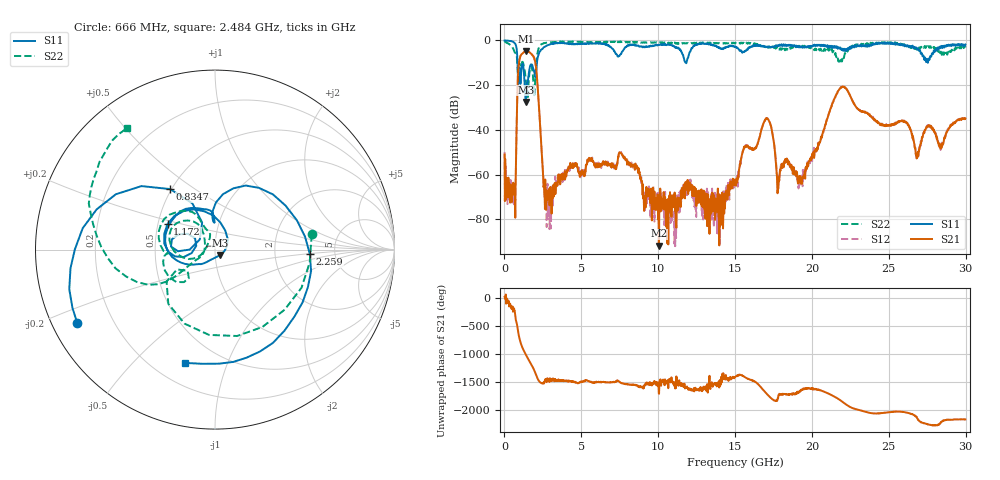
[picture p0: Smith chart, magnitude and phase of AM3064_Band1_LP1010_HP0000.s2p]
# Hz S DB R 50.0
!freq dBS11 angS11 dBS21 angS21 dBS12 angS12 dBS22 angS22
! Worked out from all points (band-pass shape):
!   1600 points, 10 MHz to 29.98 GHz, reference 50 ohm
!   highest |S21| = -4.68 dB at 1.397 GHz (marker M1); lowest = -91.9 dB at 10.04 GHz (marker M2)
!   |S21| within 3 dB of the highest: 1.011 GHz to 1.92 GHz (909.2 MHz wide, 62 % of centre)
!   lowest |S11| = -27.5 dB at 1.378 GHz (marker M3), VSWR 1.09, Z = 53 - j3.14 ohm
!   |S11| at or under -10 dB: 848.7 MHz to 2.111 GHz (1.263 GHz wide, 85.3 % of centre); 11.80178 GHz to 11.83796 GHz (36.18 MHz wide, 0.306 % of centre); 27.54303 GHz to 27.54479 GHz (1.759 MHz wide, 0.00639 % of centre)
!   |S22| runs from -26.2 to -0.3 dB; largest |S21 - S12| = 0.0077
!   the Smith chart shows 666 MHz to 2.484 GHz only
!   S11 on the Smith chart (normalised r, x): 666 MHz: 0.07, -0.25; 834.7 MHz: 0.49, +0.40; 1.172 GHz: 0.56, +0.18; 2.259 GHz: 3.23, -0.23; 2.484 GHz: 0.32, -0.72
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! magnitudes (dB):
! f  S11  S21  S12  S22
! 10 MHz  0.0  -51.1  -49.9  -0.3
! 666 MHz  -1.2  -64.9  -71.1  -5.3
! 834.7 MHz  -7.5  -24.8  -24.8  -9.8
! 1.172 GHz  -10.4  -5.9  -5.8  -9.6
! 1.378 GHz  -27.5  -4.7  -4.7  -17.1
! 1.397 GHz  -27.3  -4.7  -4.7  -18.3
! 1.959 GHz  -14.8  -8.5  -8.5  -22.3
! 2.259 GHz  -5.5  -31.2  -31.2  -2.8
! 2.484 GHz  -3.7  -56.8  -55.1  -1.6
! 2.878 GHz  -2.0  -67.5  -71.5  -0.9
! 5.015 GHz  -1.4  -59.6  -59.6  -0.6
! 7.582 GHz  -6.1  -50.4  -50.0  -0.7
! 10 GHz  -2.0  -80.1  -68.9  -1.0
! 10.04 GHz  -2.0  -91.9  -75.3  -1.0
! 15 GHz  -2.9  -63.3  -63.1  -1.4
! 17.03 GHz  -3.0  -34.8  -35.0  -3.2
! 17.82 GHz  -2.4  -66.3  -63.5  -3.5
! 19.99 GHz  -2.8  -52.3  -52.0  -3.2
! 21.94 GHz  -4.1  -21.0  -20.8  -9.5
! 25 GHz  -1.0  -38.0  -38.4  -1.1
! 26.83 GHz  -3.9  -51.9  -52.6  -3.3
! 29.98 GHz  -1.8  -34.9  -34.8  -3.2
